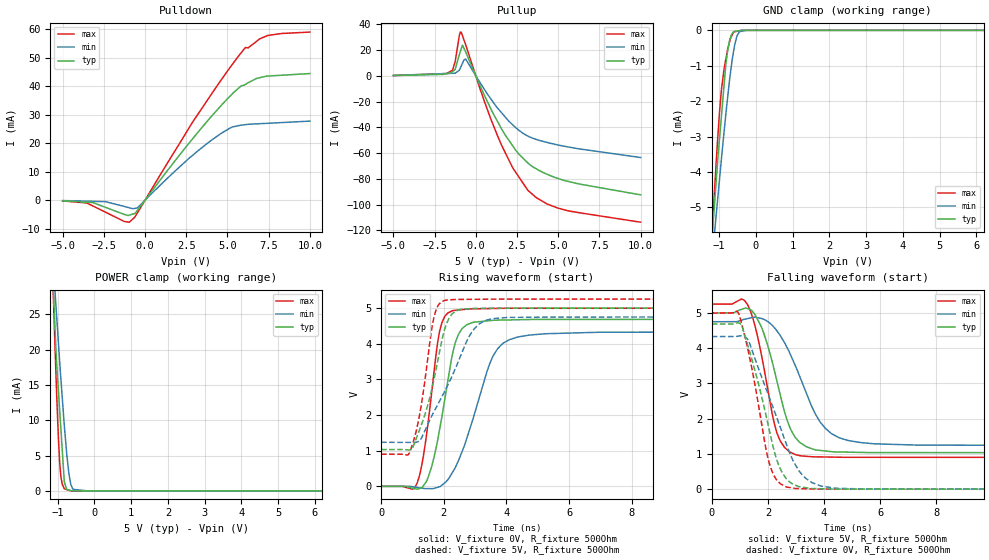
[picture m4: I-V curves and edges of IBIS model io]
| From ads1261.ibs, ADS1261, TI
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|   io Model
[Model]   io
Model_type   I/O
Polarity   Non-Inverting
Enable   Active-High
Vinl = 1.5
Vinh = 3.5
Vmeas = 2.5
Vref = 0
Cref = 4pF
Rref = 100000
|   typ   min   max
C_comp   0.704pF   0.654pF   0.741pF
|  Where Nom  PVT is Nominal Process,   5V,  27C
|   Fast PVT is Strong Process,   5.25V, -40C
|   Slow PVT is Weak Process,   4.75V, 135C
[Model spec]
|subparameter
Vinl   1.500   1.425   1.575
Vinh   3.500   3.325   3.675
[Voltage Range]   5   4.75   5.25
|Junction Temperature
[Temperature Range]   27   135   -40
[Pullup Reference]   5   4.75   5.25
[Pulldown Reference]   0   -0   0
[Power Clamp Reference]   5   4.75   5.25
[GND Clamp Reference]   0   0   0
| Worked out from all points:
|   slope of the pulldown table from 0 to 0.75 V, typ, clamps not added: 130 ohm
|   slope of the pullup table from 0 to 0.75 V, typ, clamps not added: 35.3 ohm
|   GND clamp passes 1 mA (typ) near -0.82 V on its own axis
|   POWER clamp passes 1 mA (typ) near -0.80 V on its own axis
|   falling waveform, V_fixture 5V, R_fixture 500Ohm: 20-80 % time 805ps typ, 1.17ns min, 643ps max; typ from 5 V to 1.03 V
|   rising waveform, V_fixture 0V, R_fixture 500Ohm: 20-80 % time 569ps typ, 943ps min, 424ps max; typ from 0 V to 4.68 V
|   rising waveform, V_fixture 5V, R_fixture 500Ohm: 20-80 % time 641ps typ, 1.13ns min, 434ps max; typ from 1.03 V to 5 V
|   falling waveform, V_fixture 0V, R_fixture 500Ohm: 20-80 % time 870ps typ, 1.22ns min, 689ps max; typ from 4.68 V to 0 V
[Pulldown]
|   Voltage   I(typ)   I(min)   I(max)
-5V       -239.9uA   -144uA     -282.9uA
-3.533V   -730.1uA   -360.3uA   -991.9uA
-2.405V   -2.518mA   -526.6uA   -4.216mA
-957.6mV  -5.26mA    -2.679mA   -7.742mA
-602.9mV  -4.647mA   -2.873mA   -5.803mA
-419.7mV  -3.256mA   -2.427mA   -4.039mA
1.985V    15.05mA    11.1mA     18.92mA
3.943V    28.86mA    20.7mA     36.51mA
5.295V    37.37mA    25.71mA    47.71mA
6.094V    40.69mA    26.54mA    53.66mA
7.442V    43.59mA    27mA       57.86mA
10V       44.48mA    27.77mA    59.05mA
[GND Clamp]
|   Voltage   I(typ)   I(min)   I(max)
-5V       -64.35mA   -51.58mA   -80.42mA
-1.25V    -6.695mA   -7.106mA   -6.75mA
-1.137V   -5.088mA   -5.859mA   -4.717mA
-1.053V   -3.872mA   -4.915mA   -3.27mA
-936.5mV  -2.415mA   -3.624mA   -1.67mA
-818.6mV  -975.9uA   -2.383mA   -826uA
-769.1mV  -581.7uA   -1.905mA   -544.9uA
-669.4mV  -134.5uA   -1.025mA   -174.6uA
-602.9mV  -36.14uA   -568.4uA   -51.18uA
-449.1mV  -10.42uA   -38.03uA   -12.64uA
-257.5mV  -67.38nA   -181.9nA   -123nA
10V       0A         0A         0A
[Pullup]
|   Voltage   I(typ)   I(min)   I(max)
-5V       267uA      217.6uA    282.6uA
-1.411V   3.215mA    1.972mA    4.395mA
-1.25V    5.017mA    2.051mA    11.21mA
-1.002V   16.32mA    4.329mA    31.26mA
-885.2mV  21.03mA    7.558mA    33.83mA
-800mV    23.59mA    9.997mA    30.84mA
-600.7mV  18.19mA    12.73mA    23.57mA
1.344V    -36.09mA   -25.42mA   -47.38mA
2.254V    -54.68mA   -38.24mA   -71.73mA
3.152V    -67.55mA   -46.74mA   -88.8mA
4.956V    -79.54mA   -53.61mA   -102.6mA
10V       -92.44mA   -63.43mA   -113.7mA
[POWER Clamp]
|   Voltage   I(typ)   I(min)   I(max)
-5V       589.8mA    458.4mA    751.4mA
-1.128V   29.78mA    33.13mA    29.6mA
-1.083V   24.49mA    29.36mA    22.28mA
-1.052V   20.75mA    26.69mA    17.5mA
-1.034V   18.68mA    25.33mA    14.87mA
-980mV    14.31mA    21.1mA     7.609mA
-945.2mV  11.5mA     18.4mA     4.123mA
-912.5mV  8.869mA    15.94mA    2.052mA
-817.7mV  1.293mA    9.223mA    309.2uA
-693.3mV  119.8uA    2.437mA    90.35uA
-583.2mV  1.628uA    225uA      310.2nA
10V       0A         0A         0A
[Ramp]
R_load = 500
|   typ   min   max
dV/dt_r   2.80967/5.67073e-10   2.59808/9.38323e-10   2.99626/4.2243e-10
dV/dt_f   2.38092/8.00223e-10   2.109/1.17026e-09   2.6096/6.3954e-10
[Falling Waveform]
V_fixture = 5V
V_fixture_min = 4.75V
V_fixture_max = 5.25V
R_fixture = 500Ohm
C_fixture = 0F
|   Time   V(typ)   V(min)   V(max)
0s        5V         4.75V      5.25V
1.055ns   5.099V     4.791V     5.393V
1.279ns   5.122V     4.839V     5.231V
1.769ns   4.598V     4.843V     3.809V
2.309ns   3.108V     4.504V     1.629V
2.687ns   1.948V     4.011V     1.117V
2.998ns   1.447V     3.465V     976.2mV
3.873ns   1.098V     1.894V     914.6mV
4.888ns   1.05V      1.376V     904.2mV
20ns      1.032V     1.235V     900.7mV
[Rising Waveform]
V_fixture = 0V
V_fixture_min = 0V
V_fixture_max = 0V
R_fixture = 500Ohm
C_fixture = 0F
|   Time   V(typ)   V(min)   V(max)
0s        4.65uV     6.924uV    2.998uV
1.144ns   -73.49mV   -28.8mV    74.59mV
1.301ns   -29.63mV   -49.97mV   605.9mV
1.492ns   230mV      -64.21mV   1.726V
1.859ns   1.553V     -12.6mV    4.306V
2.272ns   3.67V      381.3mV    4.92V
2.586ns   4.421V     976.5mV    4.953V
3.562ns   4.654V     3.633V     4.985V
4.337ns   4.67V      4.181V     4.992V
20ns      4.683V     4.33V      4.994V
[Rising Waveform]
V_fixture = 5V
V_fixture_min = 4.75V
V_fixture_max = 5.25V
R_fixture = 500Ohm
C_fixture = 0F
|   Time   V(typ)   V(min)   V(max)
0s        1.032V     1.235V     900.7mV
916.4ps   1.021V     1.232V     958.4mV
1.241ns   1.617V     1.286V     2.058V
1.688ns   2.995V     2.091V     4.738V
1.828ns   3.604V     2.325V     5.083V
2.034ns   4.411V     2.67V      5.215V
2.372ns   4.91V      3.305V     5.239V
2.851ns   4.983V     4.264V     5.242V
3.539ns   4.992V     4.7V       5.247V
20ns      5V         4.75V      5.25V
[Falling Waveform]
|Gnd
V_fixture = 0V
V_fixture_min = 0V
V_fixture_max = 0V
R_fixture = 500Ohm
C_fixture = 0F
|   Time   V(typ)   V(min)   V(max)
0s        4.683V     4.33V      4.994V
969.9ps   4.713V     4.343V     4.967V
1.299ns   4.034V     4.226V     3.921V
2.034ns   1.734V     2.634V     781.8mV
2.334ns   788.9mV    1.989V     242.5mV
2.661ns   293.6mV    1.268V     62.74mV
2.927ns   131.5mV    757.6mV    27.01mV
3.331ns   44.03mV    319.9mV    11.41mV
4.447ns   2.944mV    24.86mV    2.606mV
20ns      4.654uV    6.969uV    2.998uV
